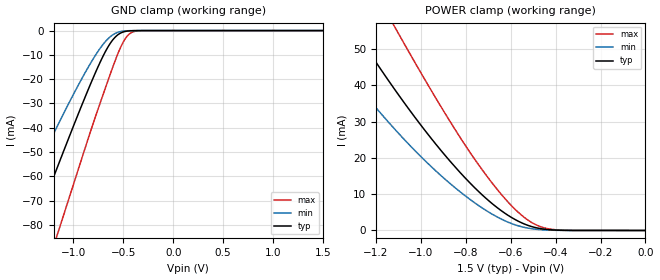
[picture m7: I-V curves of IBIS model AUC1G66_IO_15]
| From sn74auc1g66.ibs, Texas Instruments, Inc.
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[Model]   AUC1G66_IO_15
Model_type  Terminator
| variable   typ   min   max
C_comp   2.92pF   2.66pF   3.06pF
| C_tri-state   2.92pF   2.66pF   3.06pF
[Temperature Range]   40   100   -40
| Ambient temperature   25   85   -40
[Voltage range]   1.5   1.4   1.6
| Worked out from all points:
|   GND clamp passes 1 mA (typ) near -0.53 V on its own axis
|   POWER clamp passes 1 mA (typ) near -0.50 V on its own axis
[GND Clamp]
| AUC1G66_IO_15
|   Voltage   I(typ)   I(min)   I(max)
-2.7V     -221.8mA   -178.5mA   -275mA
-1.68V    -112.1mA   -84.68mA   -149.2mA
-1.635V   -107.2mA   -80.62mA   -143.6mA
-1.425V   -84.52mA   -61.93mA   -117.3mA
-1.39V    -80.75mA   -58.86mA   -112.9mA
-1.15V    -55.04mA   -38.36mA   -82.5mA
-795mV    -18.73mA   -11.15mA   -37.3mA
-670mV    -7.884mA   -4.059mA   -22.43mA
-575mV    -2.421mA   -1.028mA   -11.6mA
-475mV    -310.4uA   -114.6uA   -2.98mA
-370mV    -17.52uA   -7.845uA   -194uA
1.5V      343.9pA    9.036nA    228.6pA
[POWER Clamp]
| AUC1G66_IO_15
|   Voltage   I(typ)   I(min)   I(max)
-2.7V     212.8mA    183.5mA    242.9mA
-1.475V   73.08mA    55.64mA    96.87mA
-1.305V   56.19mA    41.71mA    77.24mA
-1.28V    53.79mA    39.77mA    74.39mA
-1.12V    39.12mA    28.13mA    56.42mA
-1.1V     37.37mA    26.77mA    54.22mA
-935mV    23.87mA    16.48mA    36.58mA
-780mV    12.99mA    8.49mA     21.35mA
-645mV    5.579mA    3.233mA    10.17mA
-540mV    1.802mA    857.8uA    3.612mA
-400mV    105.1uA    48.24uA    194.6uA
-35.59fV  343.9pA    644.5pA    263.7pA
